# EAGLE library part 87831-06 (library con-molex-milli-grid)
HEADER
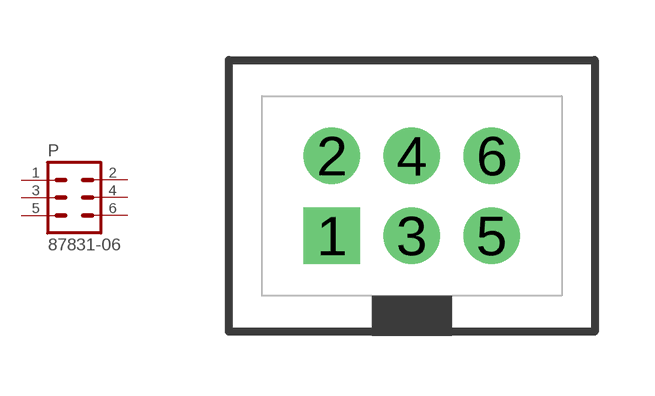
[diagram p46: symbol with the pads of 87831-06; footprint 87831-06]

Designator prefix P

## 87831-06  [87831-06]
1  1  pas
2  2  pas
3  3  pas
4  4  pas
5  5  pas
6  6  pas

## Footprint 87831-06 (pad centres in mm)
HEADER Dual Row, Shrouded, Vertical
drill 0.914 square: 1 -2,-1
drill 0.914: 2 -2,1; 3 0,-1; 4 0,1; 5 2,-1; 6 2,1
